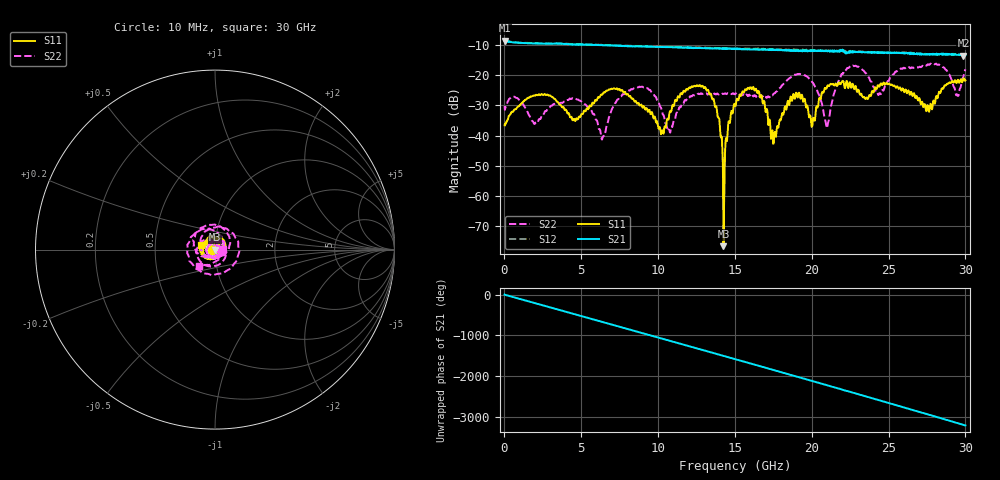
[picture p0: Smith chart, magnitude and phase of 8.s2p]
!Agilent Technologies,E8364B,US42250130,A.04.87.01
!Agilent E8364B: A.04.87.01
!Date: Monday, February 07, 2022 23:56:45
!Correction: S11(Full 2 Port SOLT,1,2) S21(Full 2 Port SOLT,1,2) S12(Full 2 Port SOLT,1,2) S22(Full 2 Port SOLT,1,2)
!S2P File: Measurements: S11, S21, S12, S22:
# Hz S  dB  R 50
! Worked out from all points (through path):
!   1601 points, 10 MHz to 30 GHz, reference 50 ohm
!   highest |S21| = -8.52 dB at 28.74 MHz (marker M1); lowest = -13.5 dB at 29.87 GHz (marker M2)
!   group delay of S21, straight-line fit = 297 ps
!   lowest |S11| = -76.7 dB at 14.26 GHz (marker M3), VSWR 1.00, Z = 50 - j0.00767 ohm
!   |S11| at or under -10 dB: start of sweep to end of sweep
!   |S22| runs from -41.3 to -16.1 dB; largest |S21 - S12| = 0.03
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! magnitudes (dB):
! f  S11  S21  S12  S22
! 10 MHz  -36.6  -8.6  -8.6  -30.2
! 28.74 MHz  -36.1  -8.5  -8.5  -31.4
! 2.147 GHz  -26.7  -9.5  -9.4  -35.7
! 5.015 GHz  -32.8  -9.9  -9.7  -28.7
! 6.42 GHz  -25.9  -10.0  -9.9  -40.3
! 7.976 GHz  -26.3  -10.3  -10.2  -25.6
! 10.02 GHz  -37.5  -10.6  -10.4  -28.7
! 10.75 GHz  -32.3  -10.7  -10.5  -38.6
! 12.98 GHz  -24.2  -11.0  -10.9  -26.1
! 13.86 GHz  -33.2  -11.1  -11.0  -26.0
! 14.26 GHz  -76.7  -11.2  -11.0  -26.2
! 15.01 GHz  -30.0  -11.2  -11.1  -26.2
! 16.43 GHz  -25.5  -11.5  -11.1  -26.8
! 17.5 GHz  -42.7  -11.5  -11.4  -26.2
! 18.9 GHz  -27.8  -11.8  -11.6  -19.8
! 20.01 GHz  -37.0  -11.7  -11.7  -22.1
! 20.98 GHz  -24.0  -12.0  -11.8  -37.5
! 22.39 GHz  -24.1  -12.3  -12.0  -17.5
! 25.01 GHz  -22.8  -12.6  -12.6  -21.8
! 27.54 GHz  -29.9  -13.1  -12.9  -16.4
! 29.87 GHz  -21.1  -13.5  -12.9  -20.5
! 30 GHz  -21.7  -13.3  -13.1  -18.0
